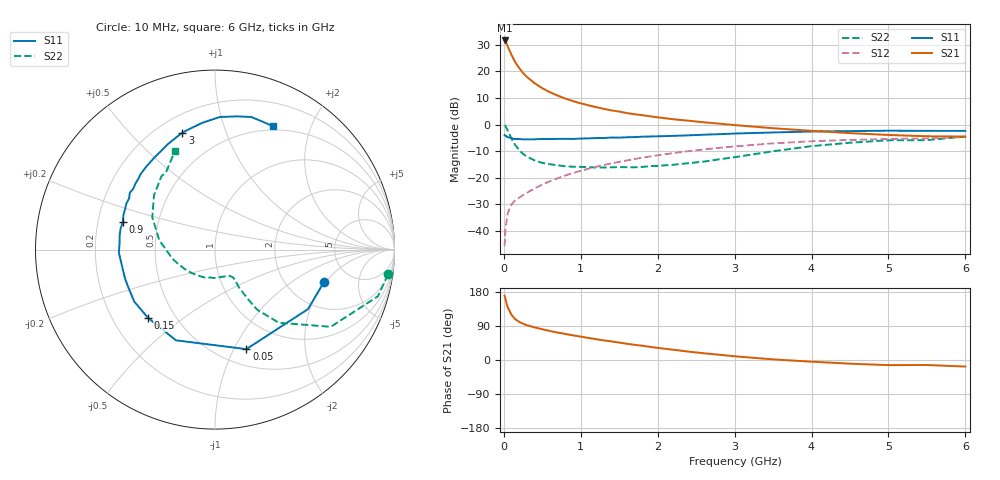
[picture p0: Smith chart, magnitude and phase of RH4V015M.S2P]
! SIEMENS Small Signal Semiconductors
! BFR106
! Si NPN RF Bipolar Junction Transistor in SOT23
! VCE = 4 V  IC = 15 mA
! Common Emitter S-Parameters:  August  1996
# GHz  S  MA  R  50
!  f  S11  S21  S12  S22
! GHz  MAG  ANG  MAG  ANG  MAG  ANG  MAG  ANG
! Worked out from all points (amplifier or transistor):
!   36 points, 10 MHz to 6 GHz, reference 50 ohm
!   highest |S21| = 31.6 dB at 10 MHz (marker M1)
!   |S21| within 3 dB of that: start of sweep to 62.52 MHz
!   unconditionally stable (mu >= 1): 406.7 MHz to 2.148 GHz; 5.407 GHz to end of sweep
!   at 250 MHz: K = 0.83, MSG = 22.9 dB, |S12| = -26.5 dB
!   at 1.4 GHz: K = 1.07, MAG = 8.3 dB, |S12| = -14.6 dB
!   at 6 GHz: K = 1.00, MAG = -0.3 dB, |S12| = -4.7 dB
!   S11 on the Smith chart (normalised r, x): 10 MHz: 3.17, -1.94; 50 MHz: 0.67, -1.12; 150 MHz: 0.35, -0.37; 900 MHz: 0.31, +0.13; 3 GHz: 0.30, +0.72; 6 GHz: 0.45, +1.47
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0.01  0.6327 -16.8  37.87 169.7  0.0052 84.2  0.9739 -8.1
0.02  0.6152 -32.6  36.21 161.3  0.0104 76.4  0.9443 -16.0
0.05  0.5814 -72.5  29.45 139.3  0.0216 61.9  0.7753 -33.7
0.1  0.5503 -113.3  20.25 119.0  0.0317 52.8  0.5408 -48.9
0.15  0.5329 -134.5  14.63 107.4  0.0378 49.9  0.4082 -55.0
0.2  0.535 -147.3  11.48 100.7  0.0424 52.1  0.3323 -56.3
0.25  0.5269 -156.0  9.286 95.6  0.0474 53.3  0.28 -57.1
0.3  0.5267 -162.4  7.825 91.9  0.0523 56.0  0.2514 -57.6
0.4  0.5275 -172.0  5.968 86.1  0.063 59.0  0.2114 -57.0
0.5  0.536 -178.2  4.8 81.1  0.0743 61.4  0.19 -56.7
0.6  0.5328 176.5  4.036 76.5  0.0863 62.9  0.1796 -58.0
0.7  0.5372 171.5  3.491 72.3  0.0979 63.8  0.1718 -60.0
0.9  0.5361 163.5  2.746 65.0  0.123 64.0  0.1611 -64.0
1.1  0.5497 155.7  2.292 58.2  0.1481 63.5  0.1585 -71.9
1.3  0.5569 149.2  1.968 51.8  0.1738 62.2  0.1558 -79.4
1.6  0.5759 140.3  1.641 42.8  0.2117 59.6  0.1581 -93.7
2.2  0.6122 124.1  1.258 27.1  0.2903 52.6  0.1754 -125.5
3  0.6768 105.6  0.976 9.8  0.3884 40.8  0.2436 -168.4
3.5  0.7093 95.9  0.852 1.6  0.4431 33.0  0.3146 170.5
4.5  0.7521 80.7  0.689 -9.7  0.5138 16.7  0.4551 138.3
5.5  0.7602 68.9  0.602 -13.2  0.5487 6.0  0.509 122.5
6  0.759 64.9  0.594 -17.3  0.5796 -1.6  0.5942 112.0
